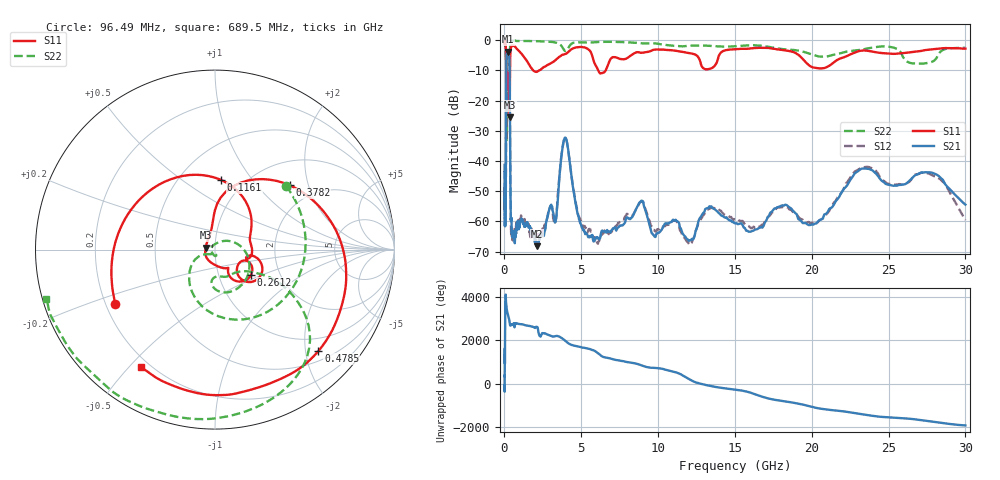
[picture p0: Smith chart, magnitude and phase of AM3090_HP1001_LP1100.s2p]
! Date/Time: Thu, Feb 28, 2019 2:03 PM
! Network Analyzer: Agilent Technologies E8364B Rev: A.07.50.67
! Sweep from 0.010 to 30.000 GHz, 1601 Points, Sweep Type: LOG
! Power Supply: 5.022 V, 0.002 A
# Hz S DB R 50
!freq MagS11 AngS11 MagS21 AngS21 MagS12 AngS12 MagS22 AngS22
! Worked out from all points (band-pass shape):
!   1601 points, 10 MHz to 30 GHz, reference 50 ohm
!   highest |S21| = -3.83 dB at 227 MHz (marker M1); lowest = -68.2 dB at 2.136 GHz (marker M2)
!   |S21| within 3 dB of the highest: 125.3 MHz to 323.9 MHz (198.6 MHz wide, 88.4 % of centre)
!   lowest |S11| = -25.5 dB at 333.7 MHz (marker M3), VSWR 1.11, Z = 45.1 + j0.896 ohm
!   |S11| at or under -10 dB: 119.7 MHz to 361 MHz (241.3 MHz wide, 100 % of centre); 1.865 GHz to 2.256 GHz (391 MHz wide, 19 % of centre); 6.099 GHz to 6.59 GHz (491.3 MHz wide, 7.74 % of centre)
!   |S22| runs from -33.6 to -0.1 dB; largest |S21 - S12| = 0.012
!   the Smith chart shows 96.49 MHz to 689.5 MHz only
!   S11 on the Smith chart (normalised r, x): 96.49 MHz: 0.24, -0.24; 116.1 MHz: 0.78, +0.72; 261.2 MHz: 1.42, -0.43; 378.2 MHz: 1.48, +1.53; 478.5 MHz: 0.70, -2.27; 689.5 MHz: 0.17, -0.54
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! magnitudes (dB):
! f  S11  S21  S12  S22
! 10 MHz  -0.3  -41.3  -43.7  -0.7
! 38.04 MHz  -0.5  -59.9  -60.8  -1.5
! 80.18 MHz  -2.0  -55.1  -55.9  -4.1
! 96.49 MHz  -4.0  -41.3  -41.2  -5.5
! 116.1 MHz  -8.2  -12.9  -13.0  -9.4
! 144.7 MHz  -14.1  -4.4  -4.4  -33.4
! 227 MHz  -16.2  -3.8  -3.8  -15.3
! 261.2 MHz  -12.2  -4.1  -4.1  -16.2
! 333.7 MHz  -25.5  -8.6  -8.6  -9.7
! 378.2 MHz  -5.2  -41.7  -40.7  -1.1
! 478.5 MHz  -1.9  -63.1  -63.8  -0.2
! 550.5 MHz  -1.9  -64.1  -66.2  -0.2
! 689.5 MHz  -2.2  -65.7  -65.3  -0.2
! 2.084 GHz  -10.5  -68.1  -64.0  -0.4
! 2.136 GHz  -10.4  -68.2  -64.6  -0.4
! 3.302 GHz  -6.7  -60.3  -60.7  -0.8
! 3.953 GHz  -4.6  -32.3  -32.3  -3.6
! 5.232 GHz  -2.5  -63.7  -61.5  -0.8
! 7.926 GHz  -6.1  -58.9  -57.8  -0.7
! 20.1 GHz  -9.1  -61.1  -60.3  -4.9
! 23.48 GHz  -3.5  -42.5  -42.0  -2.9
! 30 GHz  -2.8  -54.4  -59.5  -2.5
